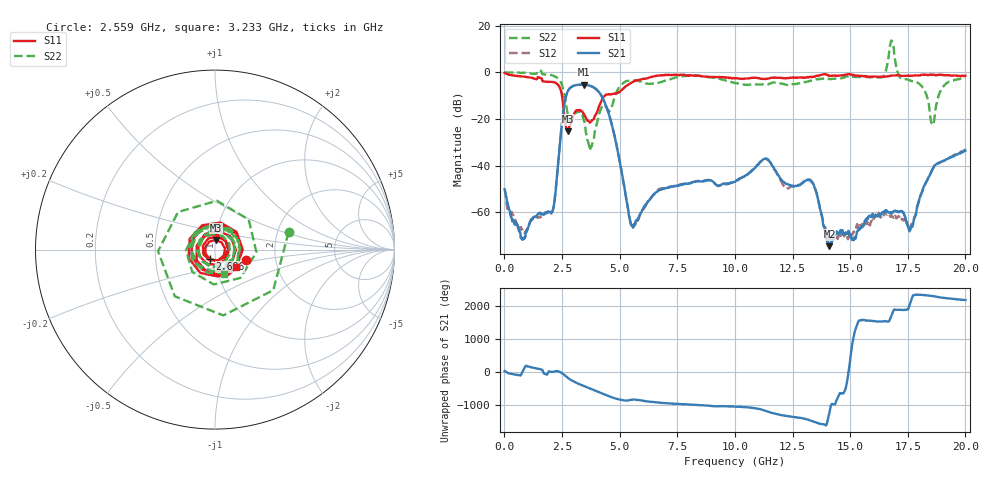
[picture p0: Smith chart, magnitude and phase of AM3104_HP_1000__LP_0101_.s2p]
!Created with skrf (http://scikit-rf.org).
# Hz S RI R 50.0
!freq ReS11 ImS11 ReS21 ImS21 ReS12 ImS12 ReS22 ImS22
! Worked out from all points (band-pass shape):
!   1601 points, 10 MHz to 20 GHz, reference 50 ohm
!   highest |S21| = -5.28 dB at 3.433 GHz (marker M1); lowest = -74.6 dB at 14.1 GHz (marker M2)
!   |S21| within 3 dB of the highest: 2.745 GHz to 4.086 GHz (1.342 GHz wide, 39.3 % of centre)
!   lowest |S11| = -25.4 dB at 2.746 GHz (marker M3), VSWR 1.11, Z = 50.1 + j5.41 ohm
!   |S11| at or under -10 dB: 2.498 GHz to 4.354 GHz (1.856 GHz wide, 54.2 % of centre)
!   |S22| runs from -33.5 to 13.6 dB; largest |S21 - S12| = 0.028
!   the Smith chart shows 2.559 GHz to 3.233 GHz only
!   S11 on the Smith chart (normalised r, x): 2.559 GHz: 1.41, -0.16; 2.696 GHz: 0.94, -0.10; 3.233 GHz: 1.25, -0.24
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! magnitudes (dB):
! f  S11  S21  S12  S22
! 10 MHz  -0.4  -50.1  -50.2  0.0
! 809.6 MHz  -1.8  -71.6  -67.9  -0.2
! 2.046 GHz  -4.1  -60.1  -60.5  -1.2
! 2.559 GHz  -14.7  -16.7  -16.8  -7.5
! 2.696 GHz  -24.4  -9.5  -9.5  -15.0
! 2.746 GHz  -25.4  -8.2  -8.2  -18.0
! 3.233 GHz  -16.3  -5.3  -5.4  -16.9
! 3.346 GHz  -16.7  -5.3  -5.4  -17.4
! 3.433 GHz  -17.8  -5.3  -5.3  -20.3
! 3.758 GHz  -21.2  -5.9  -6.0  -31.7
! 4.445 GHz  -9.5  -15.2  -15.2  -15.4
! 5.545 GHz  -4.3  -65.7  -66.3  -3.6
! 6.682 GHz  -1.4  -50.8  -50.4  -4.5
! 10.01 GHz  -2.7  -47.0  -46.8  -4.6
! 11.33 GHz  -2.9  -37.0  -37.3  -5.2
! 13.34 GHz  -2.1  -47.2  -46.9  -3.6
! 14.1 GHz  -1.5  -74.6  -71.1  -2.9
! 16.68 GHz  -1.6  -60.0  -61.3  7.2
! 17.64 GHz  -1.4  -66.3  -65.6  -3.7
! 18.56 GHz  -0.9  -41.7  -41.8  -22.2
! 19.03 GHz  -1.2  -38.1  -38.0  -6.3
! 20 GHz  -1.5  -33.6  -33.2  -2.5
